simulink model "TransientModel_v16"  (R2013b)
settings: Solver=ode4  StartTime=0.0  StopTime=1500  FixedStep=0.001  RelTol=1e-3
InitFcn:
  | Init_model
StopFcn:
  | Postprocessing2
  | %export_results
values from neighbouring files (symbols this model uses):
  dP = (0:0.005:1)'    [CurveFit_v6_trans.m]
  dP_drag = (0:0.005:1)'    [CurveFit_v6_drag.m]
  Pboost_vec_spd = n_un    [Init_steady_maps.m]
  Pboost_vec_Thr = M_un    [Init_steady_maps.m]
  Pedal = 90    [CurveFit_v6_drag.m]    (also in CurveFit_v6_trans.m = 0:10:90)
  t_sample = 0.01    [Init_model.m]
  time_dy = 0:0.01:5    [CurveFit_v6_drag.m]    (also in CurveFit_v6_trans.m = 0:0.01:10)
undefined symbols (not defined in the file or in its folder): dtaf_sub, dtMbu_sub, dtmf_sub, dtPboost_sub, dtSpeed_Turb_sub, dY, dY_af, dY_af_drag, dY_drag, dY_Mbu, dY_Mbu_drag, dY_mf, dY_mf_drag, dY_Speed_Turb, dY_Speed_Turb_drag, EngineSpeed, EngineSpeed_vec_LM, Mbu_sub_end, Mode, Pboost_Matrix, Speed, Table, Throttle_init, time_dP, time_dP_drag, time_dy_drag, Time_LM, Time_simple, Time_SM, Time_vec_LM
libraries: simulink x45, simulink_extras x4
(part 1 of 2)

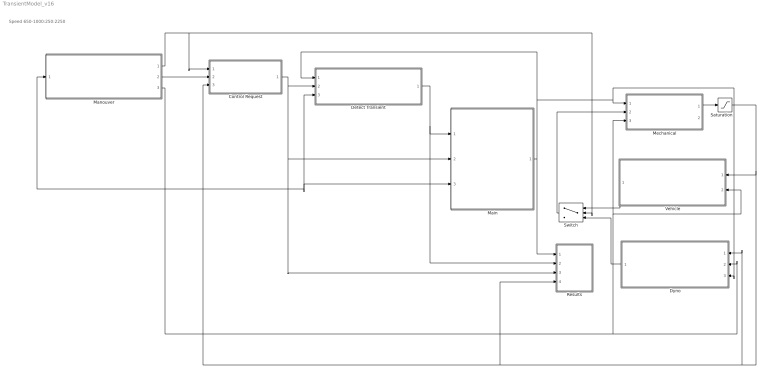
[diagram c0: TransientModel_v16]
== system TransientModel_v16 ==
  note: Speed 650-1000:250:2250
  Control Request : Subsystem
  Detect Transient : Subsystem
  Dyno : Subsystem
  Main : Subsystem
  Manouver : Subsystem
  Mechanical : Subsystem
  Results : Subsystem
  Saturation : Saturate  UpperLimit=2500  LowerLimit=650
  Switch : Switch  Threshold=3
  Vehicle : Subsystem
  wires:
  Mechanical/1(Engine_speed[1/min]) -> Saturation/1
  Switch/1 -> Mechanical/2(Mres[Nm])
  Vehicle/1(Mres[Nm]) -> Switch/1
  Dyno/1(Mdyno[Nm]) -> Switch/3
  Detect Transient/1(BUS_DetectTransient) -> Results/2(BUS_DetectTransient), Main/1(BUS_DetectTransient)
  Main/1(BUS_Main) -> Detect Transient/1(BUS_Main), Dyno/3(BUS_Main), Mechanical/1(BUS_Main), Results/1(BUS_Main)
  Control Request/1(BUS_Requests) -> Detect Transient/2(BUS_Requests), Results/3(BUS_Requests), Main/2(BUS_Requests)
  Saturation/1 -> Vehicle/1(Engine_speed[1/min]), Results/4(Engine_speed), Manouver/1(Engine Speed[1/min]), Control Request/3(Engine_speed[1/min]), Detect Transient/3(Engine_speed), Main/3(Engine Speed[1/min]), Dyno/1(Engine_speed[1/min])
  Manouver/3(Engine_Speed_dem [1/min]) -> Dyno/2(Target_speed[1/min]), Mechanical/3(Engine_speed_init[1/min]), Vehicle/2(Engine_speed_init[1/min])
  Manouver/2(Throttle_position [%]) -> Control Request/2(Throttle_position[%])
  Manouver/1(Mode [-]) -> Control Request/1(Mode[-]), Switch/2

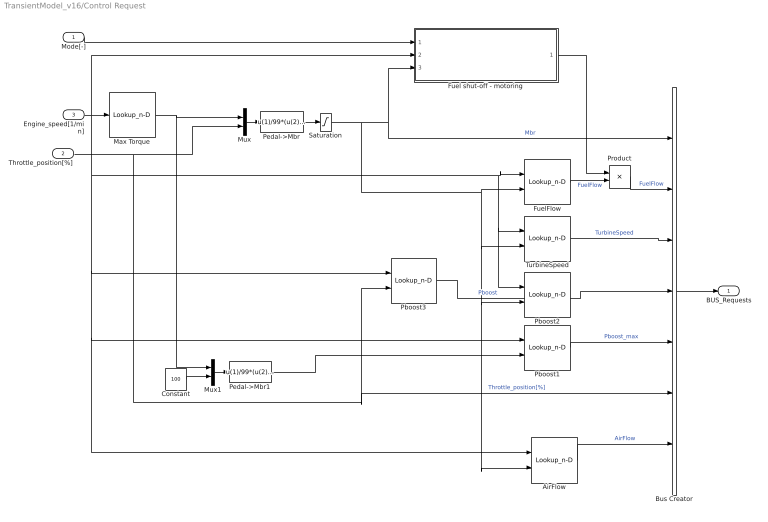
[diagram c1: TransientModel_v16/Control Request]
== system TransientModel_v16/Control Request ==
  Mode[-] : Inport
  Throttle_position[%] : Inport  Port=2
  Engine_speed[1/min] : Inport  Port=3
  AirFlow : Lookup_n-D  BreakpointsForDimension1=Table.Speed  BreakpointsForDimension2=Table.Torque  Table=Table.AirFlow  ExtrapMethod=Clip  UseLastTableValue=on  RndMeth=Simplest
  Bus Creator : BusCreator  Inputs=7
  Constant : Constant  Value=100
  Fuel shut-off - motoring : Subsystem
  FuelFlow : Lookup_n-D  BreakpointsForDimension1=Table.Speed  BreakpointsForDimension2=Table.Torque  Table=Table.FuelFlow  ExtrapMethod=Clip  UseLastTableValue=on  RndMeth=Simplest
  Max Torque : Lookup_n-D  NumberOfTableDimensions=1  BreakpointsForDimension1=|  Table=|  RndMeth=Simplest
      | [650
      | 900
      | 1300
      | 1700
      | 2100
      | 2500
      | ]
      | [400
      | 642.096
      | 868.547
      | 846.784
      | 810.772
      | 701.8]
  Mux : Mux  Inputs=2
  Mux1 : Mux  Inputs=2
  Pboost1 : Lookup_n-D  BreakpointsForDimension1=Table.Speed  BreakpointsForDimension2=Table.Torque  Table=Table.Pboost  ExtrapMethod=Clip  UseLastTableValue=on  RndMeth=Simplest
  Pboost2 : Lookup_n-D  BreakpointsForDimension1=Table.Speed  BreakpointsForDimension2=Table.Torque  Table=Table.Pboost  ExtrapMethod=Clip  UseLastTableValue=on  RndMeth=Simplest
  Pboost3 : Lookup_n-D  BreakpointsForDimension1=Pboost_vec_spd  BreakpointsForDimension2=Pboost_vec_Thr  Table=Pboost_Matrix  ExtrapMethod=Clip  UseLastTableValue=on  RndMeth=Simplest
  Pedal->Mbr : Fcn  Expr=u(1)/99*(u(2)-1)
  Pedal->Mbr1 : Fcn  Expr=u(1)/99*(u(2)-1)
  Product : Product
  Saturation : Saturate  UpperLimit=inf  LowerLimit=0
  TurbineSpeed : Lookup_n-D  BreakpointsForDimension1=Table.Speed  BreakpointsForDimension2=Table.Torque  Table=Table.SpeedTurbine  ExtrapMethod=Clip  UseLastTableValue=on  RndMeth=Simplest
  BUS_Requests : Outport
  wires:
  Mux/1 -> Pedal->Mbr/1
  Throttle_position[%]/1 -> Pboost3/2, Bus Creator/6, Mux/2  "Throttle_position[%]"
  Pedal->Mbr/1 -> Saturation/1
  Mux1/1 -> Pedal->Mbr1/1
  Max Torque/1 -> Mux1/1, Mux/1
  Constant/1 -> Mux1/2
  Pedal->Mbr1/1 -> Pboost1/2
  Pboost1/1 -> Bus Creator/5  "Pboost_max"
  Engine_speed[1/min]/1 -> Fuel shut-off - motoring/2(Engine_speed[1/min]), Max Torque/1, AirFlow/1, Pboost1/1, Pboost3/1, Pboost2/1, TurbineSpeed/1, FuelFlow/1
  Saturation/1 -> AirFlow/2, Pboost2/2, TurbineSpeed/2, FuelFlow/2, Fuel shut-off - motoring/3(Mbr [Nm]), Bus Creator/1  "Mbr"
  Bus Creator/1 -> BUS_Requests/1
  Product/1 -> Bus Creator/2  "FuelFlow"
  TurbineSpeed/1 -> Bus Creator/3  "TurbineSpeed"
  Pboost3/1 -> Bus Creator/4  "Pboost"
  FuelFlow/1 -> Product/2  "FuelFlow"
  AirFlow/1 -> Bus Creator/7  "AirFlow"
  Mode[-]/1 -> Fuel shut-off - motoring/1(Mode[-])
  Fuel shut-off - motoring/1(Fuel shut-off active [-]) -> Product/1

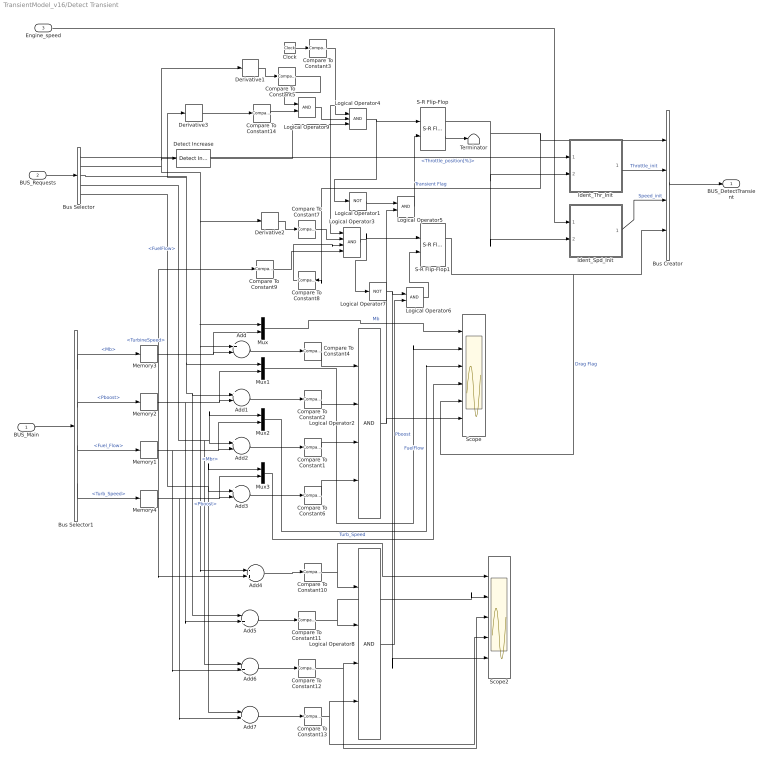
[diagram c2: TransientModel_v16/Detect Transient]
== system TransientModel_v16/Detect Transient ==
  BUS_Main : Inport
  BUS_Requests : Inport  Port=2
  Engine_speed : Inport  Port=3
  Add{,1..3} (4 alike) : Sum  Inputs=+-
  Add{4..7} (4 alike) : Sum  Inputs=-+
  Bus Creator : BusCreator
  Bus Selector : BusSelector  OutputSignals=Throttle_position[%],Mbr,Pboost,FuelFlow,TurbineSpeed
  Bus Selector1 : BusSelector  OutputSignals=Mb,Pboost,Fuel_Flow,Turb_Speed
  Clock : Clock
  Compare To Constant1 : simulink/Logic and Bit Operations/Compare To Constant  relop=<  const=0.01  OutDataTypeStr=boolean
  Compare To Constant10 : simulink/Logic and Bit Operations/Compare To Constant  relop=<  const=5  OutDataTypeStr=boolean
  Compare To Constant11 : simulink/Logic and Bit Operations/Compare To Constant  relop=<  const=0.001  OutDataTypeStr=boolean
  Compare To Constant12 : simulink/Logic and Bit Operations/Compare To Constant  relop=<  const=0.01  OutDataTypeStr=boolean
  Compare To Constant13 : simulink/Logic and Bit Operations/Compare To Constant  relop=<  const=100  OutDataTypeStr=boolean
  Compare To Constant14 : simulink/Logic and Bit Operations/Compare To Constant  relop=>=  const=0.15  OutDataTypeStr=boolean
  Compare To Constant2 : simulink/Logic and Bit Operations/Compare To Constant  relop=<  const=0.001  OutDataTypeStr=boolean
  Compare To Constant3 : simulink/Logic and Bit Operations/Compare To Constant  relop=>=  const=0.1  OutDataTypeStr=boolean
  Compare To Constant4 : simulink/Logic and Bit Operations/Compare To Constant  relop=<  const=5  OutDataTypeStr=boolean
  Compare To Constant5 : simulink/Logic and Bit Operations/Compare To Constant  relop=>=  const=50  OutDataTypeStr=boolean
  Compare To Constant6 : simulink/Logic and Bit Operations/Compare To Constant  relop=<  const=100  OutDataTypeStr=boolean
  Compare To Constant7 : simulink/Logic and Bit Operations/Compare To Constant  relop=<=  const=-50  OutDataTypeStr=boolean
  Compare To Constant8 : simulink/Logic and Bit Operations/Compare To Constant  relop===  const=0  OutDataTypeStr=boolean
  Compare To Constant9 : simulink/Logic and Bit Operations/Compare To Constant  relop=>=  const=50  OutDataTypeStr=boolean
  Derivative1 : Derivative
  Derivative2 : Derivative
  Derivative3 : Derivative
  Detect Increase : simulink/Logic and Bit Operations/Detect Increase  vinit=0.0  InputProcessing=Inherited  OutDataTypeStr=boolean
  Ident_Spd_Init : Subsystem
  Ident_Thr_Init : Subsystem
  Logical Operator1 : Logic  Operator=NOT  AllPortsSameDT=off  OutDataTypeStr=boolean
  Logical Operator2 : Logic  Inputs=4  AllPortsSameDT=off  OutDataTypeStr=boolean
  Logical Operator3 : Logic  Inputs=4  AllPortsSameDT=off  OutDataTypeStr=boolean
  Logical Operator4 : Logic  Inputs=3  AllPortsSameDT=off  OutDataTypeStr=boolean
  Logical Operator5 : Logic  AllPortsSameDT=off  OutDataTypeStr=boolean
  Logical Operator6 : Logic  AllPortsSameDT=off  OutDataTypeStr=boolean
  Logical Operator7 : Logic  Operator=NOT  AllPortsSameDT=off  OutDataTypeStr=boolean
  Logical Operator8 : Logic  Inputs=4  AllPortsSameDT=off  OutDataTypeStr=boolean
  Logical Operator9 : Logic  AllPortsSameDT=off  OutDataTypeStr=boolean
  Memory{1..4} (4 alike) : Memory
  Mux{,1..3} (4 alike) : Mux  Inputs=2
  S-R Flip-Flop : simulink_extras/Flip Flops/S-R Flip-Flop  initial_condition=0
  S-R Flip-Flop1 : simulink_extras/Flip Flops/S-R Flip-Flop  initial_condition=0
  Scope : Scope  NumInputPorts=6
  Scope2 : Scope  NumInputPorts=5
  Terminator : Terminator
  BUS_DetectTransient : Outport
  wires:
  Detect Increase/1 -> Logical Operator4/3
  Add/1 -> Compare To Constant4/1
  Bus Selector1/1 -> Memory3/1  "<Mb>"
  Bus Selector/2 -> Derivative1/1, Detect Increase/1, Mux/1, Add4/1, Add/1, Derivative2/1  "<Mbr>"
  S-R Flip-Flop/1 -> Ident_Spd_Init/2(TransientFlag), Ident_Thr_Init/2(TransientFlag), Compare To Constant8/1, Bus Creator/1  "Transient Flag"
  S-R Flip-Flop/2 -> Terminator/1
  Memory2/1 -> Add5/2, Mux1/2, Add1/2
  Add1/1 -> Compare To Constant2/1
  Bus Selector1/2 -> Memory2/1  "<Pboost>"
  Bus Selector/3 -> Derivative3/1, Add5/1, Add1/1, Mux1/1  "<Pboost>"
  Logical Operator1/1 -> Logical Operator5/1
  Logical Operator5/1 -> S-R Flip-Flop/2
  Memory3/1 -> Add4/2, Compare To Constant9/1, Mux/2, Add/2
  Clock/1 -> Compare To Constant3/1
  Logical Operator4/1 -> Logical Operator1/1, S-R Flip-Flop/1
  Compare To Constant3/1 -> Logical Operator3/1, Logical Operator4/1
  BUS_Requests/1 -> Bus Selector/1
  BUS_Main/1 -> Bus Selector1/1
  Engine_speed/1 -> Ident_Spd_Init/1(Speed)
  Bus Creator/1 -> BUS_DetectTransient/1
  Ident_Thr_Init/1(Throttle_init) -> Bus Creator/2  "Throttle_init"
  Ident_Spd_Init/1(Speed_init) -> Bus Creator/3  "Speed_init"
  Bus Selector/1 -> Ident_Thr_Init/1(Throttle)  "<Throttle_position[%]>"
  Derivative1/1 -> Compare To Constant5/1
  Bus Selector1/3 -> Memory1/1  "<Fuel_Flow>"
  Bus Selector1/4 -> Memory4/1  "<Turb_Speed>"
  Memory1/1 -> Add6/2, Mux2/2, Add2/2
  Memory4/1 -> Add7/2, Mux3/2, Add3/2
  Bus Selector/4 -> Add6/1, Mux2/1, Add2/1  "<FuelFlow>"
  Bus Selector/5 -> Add7/1, Mux3/1, Add3/1  "<TurbineSpeed>"
  Add2/1 -> Compare To Constant1/1
  Add3/1 -> Compare To Constant6/1
  Mux/1 -> Scope/1  "Mb"
  Mux1/1 -> Scope/2  "Pboost"
  Mux2/1 -> Scope/3  "FuelFlow"
  Mux3/1 -> Scope/4  "Turb_Speed"
  Compare To Constant4/1 -> Logical Operator2/1
  Compare To Constant2/1 -> Logical Operator2/2
  Compare To Constant1/1 -> Logical Operator2/3
  Compare To Constant6/1 -> Logical Operator2/4
  Logical Operator2/1 -> Logical Operator5/2, Scope/6
  Derivative2/1 -> Compare To Constant7/1
  Compare To Constant7/1 -> Logical Operator3/2
  Compare To Constant8/1 -> Logical Operator3/3
  Logical Operator3/1 -> S-R Flip-Flop1/1, Logical Operator7/1
  S-R Flip-Flop1/1 -> Scope/5, Bus Creator/4  "Drag Flag"
  Add4/1 -> Compare To Constant10/1
  Logical Operator7/1 -> Scope2/5, Logical Operator6/1
  Logical Operator6/1 -> S-R Flip-Flop1/2
  Add5/1 -> Compare To Constant11/1
  Compare To Constant10/1 -> Scope2/1, Logical Operator8/1
  Compare To Constant11/1 -> Scope2/2, Logical Operator8/2
  Add6/1 -> Compare To Constant12/1
  Compare To Constant12/1 -> Scope2/3, Logical Operator8/3
  Compare To Constant13/1 -> Scope2/4, Logical Operator8/4
  Add7/1 -> Compare To Constant13/1
  Logical Operator8/1 -> Logical Operator6/2
  Compare To Constant9/1 -> Logical Operator3/4
  Derivative3/1 -> Compare To Constant14/1
  Compare To Constant14/1 -> Logical Operator9/2
  Compare To Constant5/1 -> Logical Operator9/1
  Logical Operator9/1 -> Logical Operator4/2

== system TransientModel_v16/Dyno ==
  Engine_speed[1/min] : Inport
  Target_speed[1/min] : Inport  Port=2
  BUS_Main : Inport  Port=3
  Add : Sum  Inputs=-+
  Add1 : Sum
  Bus Selector1 : BusSelector  OutputSignals=Mb
  PID Controller : simulink/Continuous/PID Controller  Controller=PID  TimeDomain=Continuous-time  SampleTime=1  IntegratorMethod=Forward Euler  FilterMethod=Forward Euler  Form=Parallel  P=3  I=0.05  D=0  N=100  InitialConditionSource=internal  InitialConditionForIntegrator=0  InitialConditionForFilter=0  ExternalReset=none  LimitOutput=off  UpperSaturationLimit=1000  LowerSaturationLimit=0  LinearizeAsGain=off  AntiWindupMode=none  Kb=1  TrackingMode=off  Kt=1  PParamMin=[]  PParamMax=[]  IParamMin=[]  IParamMax=[]  DParamMin=[]  DParamMax=[]  NParamMin=[]  NParamMax=[]  KbParamMin=[]  KbParamMax=[]  KtParamMin=[]  KtParamMax=[]  POutMin=[]  POutMax=[]  IOutMin=[]  IOutMax=[]  DOutMin=[]  DOutMax=[]  NOutMin=[]  NOutMax=[]  KbOutMin=[]  KbOutMax=[]  KtOutMin=[]  KtOutMax=[]  IntegratorOutMin=[]  IntegratorOutMax=[]  FilterOutMin=[]  FilterOutMax=[]  SumOutMin=[]  SumOutMax=[]  SumI1OutMin=[]  SumI1OutMax=[]  SumI2OutMin=[]  SumI2OutMax=[]  SumI3OutMin=[]  SumI3OutMax=[]  SumDOutMin=[]  SumDOutMax=[]  SaturationOutMin=[]  SaturationOutMax=[]  IntegratorContinuousStateAttributes=''  IntegratorStateMustResolveToSignalObject=off  IntegratorRTWStateStorageClass=Auto  FilterContinuousStateAttributes=''  FilterStateMustResolveToSignalObject=off  FilterRTWStateStorageClass=Auto
  Mdyno[Nm] : Outport
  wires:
  Target_speed[1/min]/1 -> Add/1
  Add/1 -> PID Controller/1
  PID Controller/1 -> Add1/2
  Engine_speed[1/min]/1 -> Add/2
  Add1/1 -> Mdyno[Nm]/1
  Bus Selector1/1 -> Add1/1  "<Mb>"
  BUS_Main/1 -> Bus Selector1/1

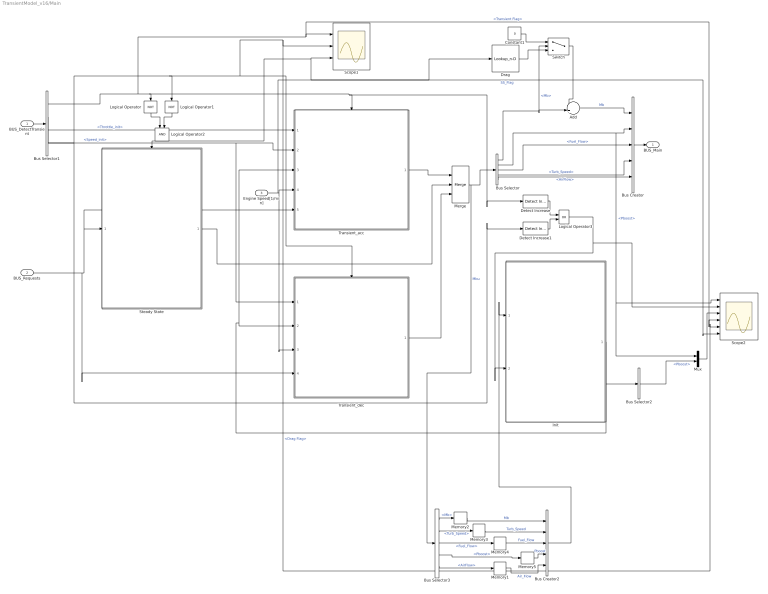
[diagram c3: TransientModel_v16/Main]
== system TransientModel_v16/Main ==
  BUS_DetectTransient : Inport
  BUS_Requests : Inport  Port=2
  Engine Speed[1/min] : Inport  Port=3
  Add : Sum
  Bus Creator : BusCreator  Inputs=5
  Bus Creator2 : BusCreator  Inputs=5
  Bus Selector : BusSelector  OutputSignals=Mb,Pboost,Fuel_Flow,Turb_Speed,AirFlow
  Bus Selector1 : BusSelector  OutputSignals=Transient Flag,Throttle_init,Speed_init,Drag Flag
  Bus Selector2 : BusSelector  OutputSignals=Pboost
  Bus Selector3 : BusSelector  OutputSignals=Mb,Turb_Speed,Fuel_Flow,Pboost,AirFlow
  Constant1 : Constant  Value=0
  Detect Increase : simulink/Logic and Bit Operations/Detect Increase  vinit=0.0  InputProcessing=Inherited  OutDataTypeStr=boolean
  Detect Increase1 : simulink/Logic and Bit Operations/Detect Increase  vinit=0.0  InputProcessing=Inherited  OutDataTypeStr=boolean
  Drag : Lookup_n-D  NumberOfTableDimensions=1  BreakpointsForDimension1="[650\t900\t1000\t1250\t1500\t1750\t2000\t2250]"  Table="[-51.7357\t-47.0411\t-45.0088\t-41.7046\t-40.0756\t-40.1524\t-41.9488\t-44.625 ]"  InternalRulePriority=Speed  RndMeth=Simplest
  Init : Subsystem  TreatAsAtomicUnit=on
  Logical Operator : Logic  Operator=NOT  AllPortsSameDT=off  OutDataTypeStr=boolean
  Logical Operator1 : Logic  Operator=NOT  AllPortsSameDT=off  OutDataTypeStr=boolean
  Logical Operator2 : Logic  AllPortsSameDT=off  OutDataTypeStr=boolean
  Logical Operator3 : Logic  Operator=OR  AllPortsSameDT=off  OutDataTypeStr=boolean
  Memory1 : Memory  X0=1
  Memory2 : Memory
  Memory3 : Memory
  Memory4 : Memory
  Memory5 : Memory  X0=1
  Merge : Merge  Inputs=3
  Mux : Mux  Inputs=2
  Scope1 : Scope  NumInputPorts=3
  Scope2 : Scope  NumInputPorts=6
  Steady State : Subsystem  TreatAsAtomicUnit=on
  Switch : Switch  Threshold=-20
  Transient_acc : Subsystem  TreatAsAtomicUnit=on
  Transient_dec : Subsystem  TreatAsAtomicUnit=on
  BUS_Main : Outport
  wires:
  Engine Speed[1/min]/1 -> Drag/1, Transient_dec/3(Speed), Transient_acc/4(Speed)
  Transient_acc/1(BUS_Transient) -> Merge/1
  Steady State/1(BUS_SS) -> Merge/2
  Merge/1 -> Bus Selector3/1, Bus Selector/1  "Mbu"
  Bus Selector/1 -> Switch/2, Add/2  "<Mb>"
  Bus Creator/1 -> BUS_Main/1
  Bus Selector/3 -> Bus Creator/3  "<Fuel_Flow>"
  Bus Selector/2 -> Scope2/1, Mux/1, Bus Creator/2  "<Pboost>"
  Bus Selector/4 -> Bus Creator/4  "<Turb_Speed>"
  BUS_Requests/1 -> Transient_dec/4(BUS_Requests), Steady State/1(BUS_Requests), Transient_acc/5(BUS_Requests)
  BUS_DetectTransient/1 -> Bus Selector1/1
  Bus Selector1/1 -> Scope2/4, Scope1/1, Detect Increase/1, Transient_acc/Enable, Logical Operator/1  "<Transient Flag>"
  Bus Selector1/2 -> Transient_acc/1(Throttle[%])  "<Throttle_init>"
  Bus Selector1/3 -> Transient_dec/1(Speed_init), Transient_acc/2(Speed_init)  "<Speed_init>"
  Bus Selector1/4 -> Detect Increase1/1, Logical Operator1/1, Scope2/5, Scope1/2, Transient_dec/Enable  "<Drag Flag>"
  Transient_dec/1(BUS_Transient) -> Merge/3
  Logical Operator1/1 -> Logical Operator2/2
  Logical Operator/1 -> Logical Operator2/1
  Logical Operator2/1 -> Steady State/Enable, Scope2/6, Scope1/3  "SS_Flag"
  Detect Increase/1 -> Logical Operator3/1
  Detect Increase1/1 -> Logical Operator3/2
  Logical Operator3/1 -> Init/2(Enable), Scope2/2
  Mux/1 -> Scope2/3
  Bus Selector3/1 -> Memory2/1  "<Mb>"
  Bus Selector3/2 -> Memory3/1  "<Turb_Speed>"
  Bus Selector3/3 -> Memory4/1  "<Fuel_Flow>"
  Bus Selector3/4 -> Memory5/1  "<Pboost>"
  Memory2/1 -> Bus Creator2/1  "Mb"
  Memory3/1 -> Bus Creator2/2  "Turb_Speed"
  Memory4/1 -> Bus Creator2/3  "Fuel_Flow"
  Memory5/1 -> Bus Creator2/4  "Pboost"
  Bus Creator2/1 -> Init/1(BUS_Requests)
  Init/1(BUS_init) -> Bus Selector2/1, Transient_dec/2(BUS_init), Transient_acc/3(BUS_init)
  Bus Selector2/1 -> Mux/2  "<Pboost>"
  Constant1/1 -> Switch/1
  Drag/1 -> Switch/3
  Add/1 -> Bus Creator/1  "Mb"
  Switch/1 -> Add/1
  Bus Selector3/5 -> Memory1/1  "<AirFlow>"
  Memory1/1 -> Bus Creator2/5  "Air_Flow"
  Bus Selector/5 -> Bus Creator/5  "<AirFlow>"

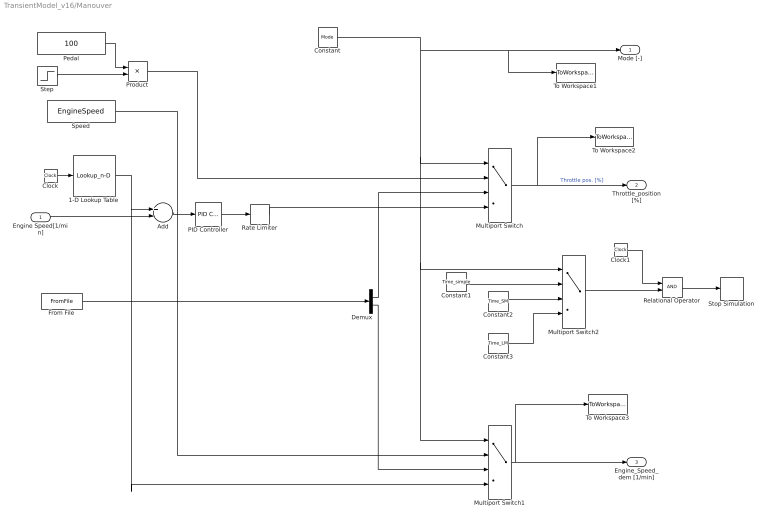
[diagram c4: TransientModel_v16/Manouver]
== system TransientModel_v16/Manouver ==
  Engine Speed[1/min] : Inport
  1-D Lookup Table : Lookup_n-D  NumberOfTableDimensions=1  BreakpointsForDimension1=Time_vec_LM  Table=EngineSpeed_vec_LM  InternalRulePriority=Speed  RndMeth=Simplest
  Add : Sum  Inputs=+-
  Clock : Clock
  Clock1 : Clock
  Constant : Constant  Value=Mode
  Constant1 : Constant  Value=Time_simple
  Constant2 : Constant  Value=Time_SM
  Constant3 : Constant  Value=Time_LM
  Demux : Demux  Outputs=2
  From File : FromFile  FileName=WHTC.mat  SampleTime=0
  Multiport Switch : MultiPortSwitch
  Multiport Switch1 : MultiPortSwitch
  Multiport Switch2 : MultiPortSwitch
  PID Controller : simulink/Continuous/PID Controller  Controller=PID  TimeDomain=Continuous-time  SampleTime=1  IntegratorMethod=Forward Euler  FilterMethod=Forward Euler  Form=Parallel  P=1  I=0.3  D=0  N=100  InitialConditionSource=internal  InitialConditionForIntegrator=25  InitialConditionForFilter=0  ExternalReset=none  LimitOutput=on  UpperSaturationLimit=100  LowerSaturationLimit=0  LinearizeAsGain=off  AntiWindupMode=clamping  Kb=1  TrackingMode=off  Kt=1  PParamMin=[]  PParamMax=[]  IParamMin=[]  IParamMax=[]  DParamMin=[]  DParamMax=[]  NParamMin=[]  NParamMax=[]  KbParamMin=[]  KbParamMax=[]  KtParamMin=[]  KtParamMax=[]  POutMin=[]  POutMax=[]  IOutMin=[]  IOutMax=[]  DOutMin=[]  DOutMax=[]  NOutMin=[]  NOutMax=[]  KbOutMin=[]  KbOutMax=[]  KtOutMin=[]  KtOutMax=[]  IntegratorOutMin=[]  IntegratorOutMax=[]  FilterOutMin=[]  FilterOutMax=[]  SumOutMin=[]  SumOutMax=[]  SumI1OutMin=[]  SumI1OutMax=[]  SumI2OutMin=[]  SumI2OutMax=[]  SumI3OutMin=[]  SumI3OutMax=[]  SumDOutMin=[]  SumDOutMax=[]  SaturationOutMin=[]  SaturationOutMax=[]  IntegratorContinuousStateAttributes=''  IntegratorStateMustResolveToSignalObject=off  IntegratorRTWStateStorageClass=Auto  FilterContinuousStateAttributes=''  FilterStateMustResolveToSignalObject=off  FilterRTWStateStorageClass=Auto
  Pedal : Constant  Value=100
  Product : Product
  Rate Limiter : RateLimiter  RisingSlewLimit=inf  FallingSlewLimit=-200  SampleTimeMode=inherited
  Relational Operator : RelationalOperator  OutDataTypeStr=boolean
  Speed : Constant  Value=EngineSpeed
  Step : Step  Time=5  Before=Throttle_init/100  SampleTime=0
  Stop Simulation : Stop
  To Workspace1 : ToWorkspace  VariableName=Mode  SampleTime=-1
  To Workspace2 : ToWorkspace  VariableName=Pedal_set  SampleTime=-1
  To Workspace3 : ToWorkspace  VariableName=Speed_set  SampleTime=-1
  Mode [-] : Outport
  Throttle_position [%] : Outport  Port=2
  Engine_Speed_dem [1/min] : Outport  Port=3
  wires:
  Step/1 -> Product/2
  Pedal/1 -> Product/1
  Multiport Switch1/1 -> Engine_Speed_dem [1/min]/1, To Workspace3/1
  From File/1 -> Demux/1
  Demux/1 -> Multiport Switch/3
  Demux/2 -> Multiport Switch1/3
  Add/1 -> PID Controller/1
  Clock/1 -> 1-D Lookup Table/1
  1-D Lookup Table/1 -> Multiport Switch1/4, Add/1
  PID Controller/1 -> Rate Limiter/1
  Engine Speed[1/min]/1 -> Add/2
  Product/1 -> Multiport Switch/2
  Rate Limiter/1 -> Multiport Switch/4
  Speed/1 -> Multiport Switch1/2
  Multiport Switch/1 -> Throttle_position [%]/1, To Workspace2/1  "Throttle pos. [%]"
  Constant/1 -> To Workspace1/1, Mode [-]/1, Multiport Switch/1, Multiport Switch1/1, Multiport Switch2/1
  Constant1/1 -> Multiport Switch2/2
  Constant2/1 -> Multiport Switch2/3
  Constant3/1 -> Multiport Switch2/4
  Clock1/1 -> Relational Operator/1
  Multiport Switch2/1 -> Relational Operator/2
  Relational Operator/1 -> Stop Simulation/1

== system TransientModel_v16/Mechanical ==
  BUS_Main : Inport
  Mres[Nm] : Inport  Port=2
  Engine_speed_init[1/min] : Inport  Port=3
  Add1 : Sum  Inputs=+-
  Bus Selector1 : BusSelector  OutputSignals=Mb
  Gain : Gain  Gain=1/1.2
  Gain1 : Gain  Gain=pi/30
  Integrator : Integrator  InitialConditionSource=external  InitialCondition=2000/30*pi
  Product : Product
  rad2rpm1 : Gain  Gain=30/pi
  Engine_speed[1/min] : Outport
  Pemech : Outport  Port=2
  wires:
  Product/1 -> Pemech/1
  Integrator/1 -> Product/1, rad2rpm1/1  "om_e"
  Gain/1 -> Integrator/1
  Add1/1 -> Gain/1
  rad2rpm1/1 -> Engine_speed[1/min]/1
  Mres[Nm]/1 -> Add1/2
  Engine_speed_init[1/min]/1 -> Gain1/1
  Gain1/1 -> Integrator/2
  Bus Selector1/1 -> Add1/1, Product/2  "<Mb>"
  BUS_Main/1 -> Bus Selector1/1

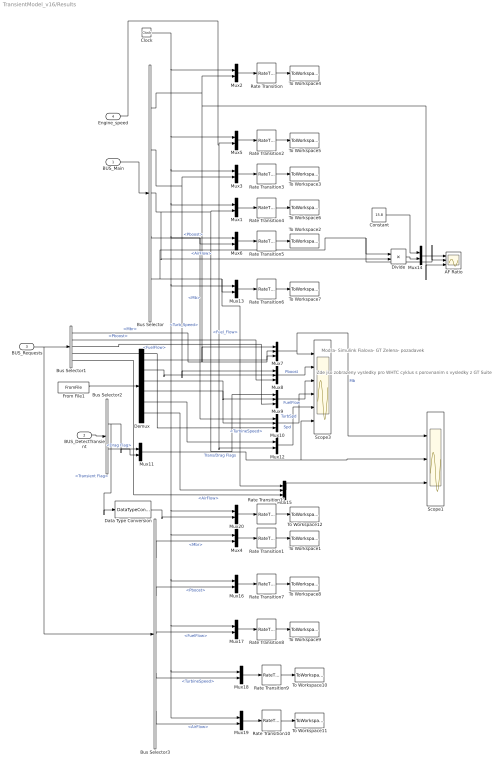
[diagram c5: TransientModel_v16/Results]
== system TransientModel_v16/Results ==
  note: Zde jso zobrazeny vysledky pro WHTC cyklus s porovnanim s vysledky z GT Suite
  note: Modra- Simulink Fialova- GT Zelena- pozadavek
  BUS_Main : Inport
  BUS_DetectTransient : Inport  Port=2
  BUS_Requests : Inport  Port=3
  Engine_speed : Inport  Port=4
  AF Ratio : Scope  NumInputPorts=3
  Bus Selector : BusSelector  OutputSignals=Mb,Pboost,Fuel_Flow,Turb_Speed,AirFlow
  Bus Selector1 : BusSelector  OutputSignals=Mbr,Pboost,FuelFlow,TurbineSpeed,AirFlow
  Bus Selector2 : BusSelector  OutputSignals=Transient Flag,Drag Flag
  Bus Selector3 : BusSelector  OutputSignals=Mbr,Pboost,FuelFlow,TurbineSpeed,AirFlow
  Clock : Clock
  Constant : Constant  Value=15.8
  Data Type Conversion : DataTypeConversion
  Demux : Demux  Outputs=6
  Divide : Product  Inputs=*/
  From File1 : FromFile  FileName=GT_WHTC_speed2.mat  SampleTime=0
  Mux{1..6,11..14,16..20} (15 alike) : Mux  Inputs=2
  Mux{7..10,15} (5 alike) : Mux  Inputs=3
  Rate Transition{,1..11} (12 alike) : RateTransition
  Scope1 : Scope  NumInputPorts=3
  Scope3 : Scope  NumInputPorts=6
  To Workspace1 : ToWorkspace  VariableName=Sim2GT_Mbr  SampleTime=t_sample
  To Workspace10 : ToWorkspace  VariableName=Sim2GT_TurbSpeed_r  SampleTime=t_sample
  To Workspace11 : ToWorkspace  VariableName=Sim2GT_AirFlow_r  SampleTime=t_sample
  To Workspace12 : ToWorkspace  VariableName=Sim2GT_Trans_Flag  SampleTime=t_sample
  To Workspace2 : ToWorkspace  VariableName=Sim2GT_TurbSpeed  SampleTime=t_sample
  To Workspace3 : ToWorkspace  VariableName=Sim2GT_Pboost  SampleTime=t_sample
  To Workspace4 : ToWorkspace  VariableName=Sim2GT_Mb  SampleTime=t_sample
  To Workspace5 : ToWorkspace  VariableName=Sim2GT_speed  SampleTime=t_sample
  To Workspace6 : ToWorkspace  VariableName=Sim2GT_Mb_FuelFlow  SampleTime=t_sample
  To Workspace7 : ToWorkspace  VariableName=Sim2GT_AirFlow  SampleTime=t_sample
  To Workspace8 : ToWorkspace  VariableName=Sim2GT_Pboost_r  SampleTime=t_sample
  To Workspace9 : ToWorkspace  VariableName=Sim2GT_Mb_FuelFlow_r  SampleTime=t_sample
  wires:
  Rate Transition/1 -> To Workspace4/1
  Mux2/1 -> Rate Transition/1
  Rate Transition2/1 -> To Workspace5/1
  Mux5/1 -> Rate Transition2/1
  Rate Transition3/1 -> To Workspace3/1
  Mux3/1 -> Rate Transition3/1
  Bus Selector1/1 -> Mux7/3  "<Mbr>"
  Engine_speed/1 -> Mux12/2, Mux5/2
  Bus Selector/2 -> Mux8/1, Mux3/2  "<Pboost>"
  BUS_Main/1 -> Bus Selector/1
  Bus Selector/1 -> AF Ratio/3, Mux7/1, Mux2/2  "<Mb>"
  Clock/1 -> Mux2/1, Mux5/1, Mux19/1, Mux18/1, Mux17/1, Mux16/1, Mux4/1, Mux20/1, Mux13/1, Mux6/1, Mux1/1, Mux3/1
  Rate Transition4/1 -> To Workspace6/1
  Mux1/1 -> Rate Transition4/1
  Rate Transition5/1 -> To Workspace2/1
  Mux6/1 -> Rate Transition5/1
  Bus Selector/4 -> Mux10/1, Mux6/2  "<Turb_Speed>"
  Bus Selector/3 -> Divide/2, Mux9/1, Mux1/2  "<Fuel_Flow>"
  From File1/1 -> Demux/1
  Demux/1 -> Mux7/2
  Mux7/1 -> Scope1/1, Scope3/1  "Mb"
  Mux8/1 -> Scope3/2  "Pboost"
  Mux9/1 -> Scope3/3  "FuelFlow"
  Mux10/1 -> Scope3/4  "TurbSpd"
  Demux/2 -> Mux8/2
  Demux/3 -> Mux9/2
  Demux/4 -> Mux10/2
  Bus Selector1/2 -> Mux8/3  "<Pboost>"
  BUS_Requests/1 -> Bus Selector3/1, Bus Selector1/1
  BUS_DetectTransient/1 -> Bus Selector2/1
  Bus Selector2/1 -> Data Type Conversion/1, Mux11/1  "<Transient Flag>"
  Bus Selector2/2 -> Mux11/2  "<Drag Flag>"
  Demux/5 -> Mux12/1
  Mux12/1 -> Scope3/5  "Spd"
  Mux11/1 -> Scope1/2, Scope3/6  "Trans/Drag Flags"
  Bus Selector1/3 -> Mux9/3  "<FuelFlow>"
  Bus Selector1/4 -> Mux10/3  "<TurbineSpeed>"
  Bus Selector/5 -> AF Ratio/2, Divide/1, Mux15/1, Mux13/2  "<AirFlow>"
  Mux13/1 -> Rate Transition6/1
  Rate Transition6/1 -> To Workspace7/1
  Mux14/1 -> AF Ratio/1
  Divide/1 -> Mux14/2
  Constant/1 -> Mux14/1
  Demux/6 -> Mux15/2
  Bus Selector1/5 -> Mux15/3  "<AirFlow>"
  Mux15/1 -> Scope1/3
  Rate Transition7/1 -> To Workspace8/1
  Mux16/1 -> Rate Transition7/1
  Bus Selector3/2 -> Mux16/2  "<Pboost>"
  Rate Transition8/1 -> To Workspace9/1
  Mux17/1 -> Rate Transition8/1
  Bus Selector3/3 -> Mux17/2  "<FuelFlow>"
  Rate Transition9/1 -> To Workspace10/1
  Mux18/1 -> Rate Transition9/1
  Bus Selector3/4 -> Mux18/2  "<TurbineSpeed>"
  Rate Transition1/1 -> To Workspace1/1
  Mux4/1 -> Rate Transition1/1
  Bus Selector3/1 -> Mux4/2  "<Mbr>"
  Mux19/1 -> Rate Transition10/1
  Rate Transition10/1 -> To Workspace11/1
  Bus Selector3/5 -> Mux19/2  "<AirFlow>"
  Rate Transition11/1 -> To Workspace12/1
  Mux20/1 -> Rate Transition11/1
  Data Type Conversion/1 -> Mux20/2

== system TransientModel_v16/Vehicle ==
  Engine_speed[1/min] : Inport
  Engine_speed_init[1/min] : Inport  Port=2
  Add4 : Sum  Inputs=+-
  Add5 : Sum
  Driving resistance : Lookup_n-D  NumberOfTableDimensions=1  BreakpointsForDimension1=|  Table=|  ExtrapMethod=Clip  RndMeth=Simplest
      | [650
      | 900
      | 1000
      | 1100
      | 1200
      | 1300
      | 1400
      | 1500
      | 1600
      | 1700
      | 1800
      | 1900
      | 2000
      | 2100
      | 2200
      | 2300
      | 2400
      | 2500
      | 2600
      | 2700]
      | [140.201383
      | 153.6645939
      | 160.2659102
      | 167.5621018
      | 175.5531689
      | 184.2391114
      | 193.6199293
      | 203.6956225
      | 214.4661912
      | 225.9316353
      | 238.0919548
      | 250.9471496
      | 264.4972199
      | 278.7421655
      | 293.6819866
      | 309.3166831
      | 325.6462549
      | 342.6707022
      | 360.3900248
      | 378.8042229]
  Gain1 : Gain  Gain=pi/30
  Idle_gear & Blocker Ring : Gain  Gain=1/74.4
  Integrator1 : Integrator  InitialConditionSource=external  InitialCondition=900/30*pi
  Integrator3 : Integrator
  Sum : Sum  Inputs=+-
  b_cg : Gain  Gain=5
  k_cg : Gain  Gain=2500000
  n2rad : Gain  Gain=pi/30
  rad2rpm : Gain  Gain=30/pi
  Mres[Nm] : Outport
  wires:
  b_cg/1 -> Add5/2
  k_cg/1 -> Add5/1
  Integrator3/1 -> k_cg/1
  Add4/1 -> Integrator3/1, b_cg/1
  Idle_gear & Blocker Ring/1 -> Integrator1/1
  Sum/1 -> Idle_gear & Blocker Ring/1
  Integrator1/1 -> rad2rpm/1, Add4/2
  rad2rpm/1 -> Driving resistance/1
  Engine_speed[1/min]/1 -> n2rad/1
  n2rad/1 -> Add4/1
  Driving resistance/1 -> Sum/2
  Add5/1 -> Mres[Nm]/1, Sum/1
  Engine_speed_init[1/min]/1 -> Gain1/1
  Gain1/1 -> Integrator1/2

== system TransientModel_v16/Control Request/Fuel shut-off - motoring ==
  Mode[-] : Inport
  Engine_speed[1/min] : Inport  Port=2
  Mbr [Nm] : Inport  Port=3
  0 : Constant  Value=0
  1 : Constant
  Compare To Constant : simulink/Logic and Bit Operations/Compare To Constant  relop=<=  const=0  OutDataTypeStr=boolean
  Fuel-shut-off : Switch  Threshold=3
  Fuel-shut-off rpm : simulink/Logic and Bit Operations/Compare To Constant  relop=>=  const=900  OutDataTypeStr=boolean
  Logical Operator : Logic  Operator=NAND  Inputs=3  AllPortsSameDT=off  OutDataTypeStr=boolean
  Fuel shut-off active [-] : Outport
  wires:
  Compare To Constant/1 -> Logical Operator/1
  Fuel-shut-off rpm/1 -> Logical Operator/2
  Logical Operator/1 -> Fuel shut-off active [-]/1
  Fuel-shut-off/1 -> Logical Operator/3
  Mbr [Nm]/1 -> Compare To Constant/1
  Engine_speed[1/min]/1 -> Fuel-shut-off rpm/1
  1/1 -> Fuel-shut-off/1
  0/1 -> Fuel-shut-off/3
  Mode[-]/1 -> Fuel-shut-off/2

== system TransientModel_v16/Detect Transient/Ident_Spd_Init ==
  Speed : Inport
  TransientFlag : Inport  Port=2
  Clock : Clock
  Compare To Constant : simulink/Logic and Bit Operations/Compare To Constant  relop=>=  const=0.1  OutDataTypeStr=uint8
  Detect Increase : simulink/Logic and Bit Operations/Detect Increase  vinit=0.0  InputProcessing=Inherited  OutDataTypeStr=uint8
  Enabled Subsystem : Subsystem  TreatAsAtomicUnit=on
  Logical Operator : Logic  AllPortsSameDT=off  OutDataTypeStr=boolean
  Memory : Memory
  Memory1 : Memory
  S-R Flip-Flop : simulink_extras/Flip Flops/S-R Flip-Flop  initial_condition=0
  Switch : Switch
  Speed_init : Outport
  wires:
  TransientFlag/1 -> Detect Increase/1
  Memory1/1 -> Enabled Subsystem/1(In1)
  Memory/1 -> Switch/1
  Enabled Subsystem/1(Out1) -> Switch/3
  Switch/1 -> Speed_init/1, Memory1/1
  Compare To Constant/1 -> Logical Operator/2
  Clock/1 -> Compare To Constant/1
  Logical Operator/1 -> Switch/2, S-R Flip-Flop/1
  Detect Increase/1 -> Logical Operator/1
  S-R Flip-Flop/1 -> Enabled Subsystem/Enable
  Speed/1 -> Memory/1

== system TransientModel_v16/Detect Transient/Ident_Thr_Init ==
  Throttle : Inport
  TransientFlag : Inport  Port=2
  Clock : Clock
  Compare To Constant : simulink/Logic and Bit Operations/Compare To Constant  relop=>=  const=0.1  OutDataTypeStr=uint8
  Detect Increase : simulink/Logic and Bit Operations/Detect Increase  vinit=0.0  InputProcessing=Inherited  OutDataTypeStr=uint8
  Enabled Subsystem : Subsystem  TreatAsAtomicUnit=on
  Logical Operator : Logic  AllPortsSameDT=off  OutDataTypeStr=boolean
  Memory : Memory
  Memory1 : Memory
  S-R Flip-Flop : simulink_extras/Flip Flops/S-R Flip-Flop  initial_condition=0
  Switch : Switch
  Throttle_init : Outport
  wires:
  Throttle/1 -> Memory/1
  S-R Flip-Flop/1 -> Enabled Subsystem/Enable
  Detect Increase/1 -> Logical Operator/1
  Logical Operator/1 -> S-R Flip-Flop/1, Switch/2
  Clock/1 -> Compare To Constant/1
  Compare To Constant/1 -> Logical Operator/2
  Switch/1 -> Memory1/1, Throttle_init/1
  Enabled Subsystem/1(Out1) -> Switch/3
  Memory/1 -> Switch/1
  Memory1/1 -> Enabled Subsystem/1(In1)
  TransientFlag/1 -> Detect Increase/1

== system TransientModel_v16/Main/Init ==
  BUS_Requests : Inport
  Enable : Inport  Port=2
  Subsystem : Subsystem
  BUS_init : Outport
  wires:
  BUS_Requests/1 -> Subsystem/1(In1)
  Enable/1 -> Subsystem/Enable
  Subsystem/1(Out1) -> BUS_init/1

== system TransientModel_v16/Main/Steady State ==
  BUS_Requests : Inport
  Enable : EnablePort
  Bus Creator1 : BusCreator  Inputs=5
  Bus Selector : BusSelector  OutputSignals=Mbr,TurbineSpeed,FuelFlow,Pboost,AirFlow
  Gain{,1..4} (5 alike) : Gain
  Memory{1..5} (5 alike) : Memory
  BUS_SS : Outport
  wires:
  Bus Selector/2 -> Memory3/1, Gain1/1  "<TurbineSpeed>"
  Bus Selector/3 -> Gain2/1, Memory1/1  "<FuelFlow>"
  Bus Selector/4 -> Gain3/1, Memory4/1  "<Pboost>"
  Bus Creator1/1 -> BUS_SS/1
  Gain/1 -> Bus Creator1/2  "Mb"
  Gain3/1 -> Bus Creator1/1  "Pboost"
  Gain2/1 -> Bus Creator1/3  "Fuel_Flow"
  Gain1/1 -> Bus Creator1/4  "Turb_Speed"
  BUS_Requests/1 -> Bus Selector/1
  Bus Selector/1 -> Memory2/1, Gain/1  "<Mbr>"
  Bus Selector/5 -> Memory5/1, Gain4/1  "<AirFlow>"
  Gain4/1 -> Bus Creator1/5  "AirFlow"

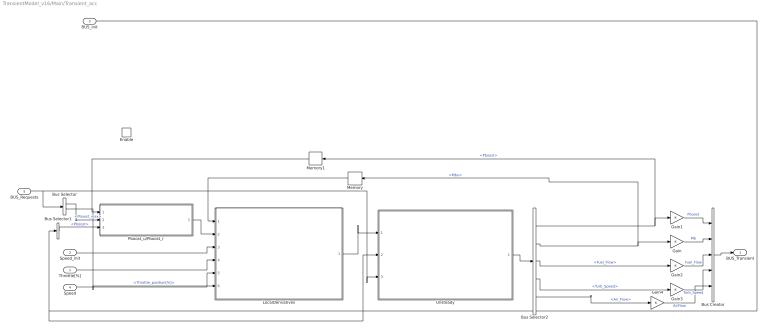
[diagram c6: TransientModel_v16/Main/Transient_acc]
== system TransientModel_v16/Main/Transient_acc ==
  Throttle[%] : Inport
  Speed_init : Inport  Port=2
  BUS_init : Inport  Port=3
  Speed : Inport  Port=4
  BUS_Requests : Inport  Port=5
  Enable : EnablePort  StatesWhenEnabling=reset
  Bus Creator : BusCreator  Inputs=5
  Bus Selector : BusSelector  OutputSignals=Pboost_max,Throttle_position[%]
  Bus Selector1 : BusSelector  OutputSignals=Pboost
  Bus Selector2 : BusSelector  OutputSignals=Pboost,Mbu,Fuel_Flow,Turb_Speed,Air_Flow
  Gain{,1..4} (5 alike) : Gain
  LocalDerivatives : Subsystem
  Memory : Memory
  Memory1 : Memory
  Pboost_u/Pboost_r : Subsystem
  Unsteady : Subsystem
  BUS_Transient : Outport
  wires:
  Bus Creator/1 -> BUS_Transient/1
  Gain1/1 -> Bus Creator/1  "Pboost"
  Gain/1 -> Bus Creator/2  "Mb"
  Gain2/1 -> Bus Creator/3  "Fuel_Flow"
  Gain3/1 -> Bus Creator/4  "Turb_Speed"
  Speed/1 -> LocalDerivatives/5(Speed)
  Speed_init/1 -> LocalDerivatives/3(Speed_init)
  Throttle[%]/1 -> LocalDerivatives/4(Throttle_init[%])
  Pboost_u/Pboost_r/1(Pboost_u/Pboost_r) -> LocalDerivatives/2(Pboost_u/Pboost_r)
  Bus Selector1/1 -> Pboost_u/Pboost_r/3(Pboost_init)  "<Pboost>"
  LocalDerivatives/1(BUS_Derivatives) -> Unsteady/1(BUS_Derivatives)
  Unsteady/1(BUS_Unsteady) -> Bus Selector2/1
  Bus Selector2/2 -> Memory/1, Gain/1  "<Mbu>"
  Bus Selector2/1 -> Memory1/1, Gain1/1  "<Pboost>"
  Bus Selector2/3 -> Gain2/1  "<Fuel_Flow>"
  Bus Selector2/4 -> Gain3/1  "<Turb_Speed>"
  Memory/1 -> LocalDerivatives/1(Mbu)
  Memory1/1 -> Pboost_u/Pboost_r/1(Pboost_u)
  BUS_Requests/1 -> Bus Selector/1, Unsteady/3(BUS_Requests)
  Bus Selector/1 -> Pboost_u/Pboost_r/2(Pboostr_max[bar])  "<Pboost_max>"
  BUS_init/1 -> Bus Selector1/1, Unsteady/2(BUS_init)
  Gain4/1 -> Bus Creator/5  "AirFlow"
  Bus Selector2/5 -> Gain4/1  "<Air_Flow>"
  Bus Selector/2 -> LocalDerivatives/6(Throttle_act[%])  "<Throttle_position[%]>"

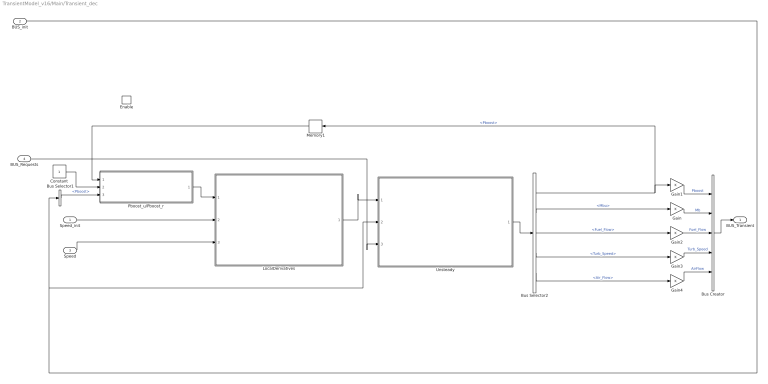
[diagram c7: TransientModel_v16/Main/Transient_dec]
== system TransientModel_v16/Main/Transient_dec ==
  Speed_init : Inport
  BUS_init : Inport  Port=2
  Speed : Inport  Port=3
  BUS_Requests : Inport  Port=4
  Enable : EnablePort  StatesWhenEnabling=reset
  Bus Creator : BusCreator  Inputs=5
  Bus Selector1 : BusSelector  OutputSignals=Pboost
  Bus Selector2 : BusSelector  OutputSignals=Pboost,Mbu,Fuel_Flow,Turb_Speed,Air_Flow
  Constant : Constant
  Gain{,1..4} (5 alike) : Gain
  LocalDerivatives : Subsystem
  Memory1 : Memory
  Pboost_u/Pboost_r : Subsystem
  Unsteady : Subsystem
  BUS_Transient : Outport
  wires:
  BUS_Requests/1 -> Unsteady/3(BUS_Requests)
  Memory1/1 -> Pboost_u/Pboost_r/1(Pboost_u)
  Bus Selector2/4 -> Gain3/1  "<Turb_Speed>"
  Bus Selector2/3 -> Gain2/1  "<Fuel_Flow>"
  Bus Selector2/1 -> Gain1/1, Memory1/1  "<Pboost>"
  Bus Selector2/2 -> Gain/1  "<Mbu>"
  Unsteady/1(BUS_Unsteady) -> Bus Selector2/1
  LocalDerivatives/1(BUS_Derivatives) -> Unsteady/1(BUS_Derivatives)
  Bus Selector1/1 -> Pboost_u/Pboost_r/3(Pboost_init)  "<Pboost>"
  Pboost_u/Pboost_r/1(Pboost_u/Pboost_r) -> LocalDerivatives/1(Pboost_u/Pboost_r)
  Speed_init/1 -> LocalDerivatives/2(Speed_init)
  Speed/1 -> LocalDerivatives/3(Speed)
  Gain3/1 -> Bus Creator/4  "Turb_Speed"
  Gain2/1 -> Bus Creator/3  "Fuel_Flow"
  Gain/1 -> Bus Creator/2  "Mb"
  Gain1/1 -> Bus Creator/1  "Pboost"
  BUS_init/1 -> Bus Selector1/1, Unsteady/2(BUS_init)
  Bus Creator/1 -> BUS_Transient/1
  Constant/1 -> Pboost_u/Pboost_r/2(Pboostr_max[bar])
  Gain4/1 -> Bus Creator/5  "AirFlow"
  Bus Selector2/5 -> Gain4/1  "<Air_Flow>"

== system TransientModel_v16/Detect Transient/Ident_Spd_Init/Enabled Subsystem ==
  In1 : Inport
  Enable : EnablePort
  Out1 : Outport
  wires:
  In1/1 -> Out1/1

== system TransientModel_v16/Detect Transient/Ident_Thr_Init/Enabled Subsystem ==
  In1 : Inport
  Enable : EnablePort
  Out1 : Outport
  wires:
  In1/1 -> Out1/1

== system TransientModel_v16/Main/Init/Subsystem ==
  In1 : Inport
  Enable : EnablePort
  Bus Creator2 : BusCreator  Inputs=5
  Bus Selector : BusSelector  OutputSignals=Mb,Turb_Speed,Fuel_Flow,Pboost,Air_Flow
  Out1 : Outport
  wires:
  In1/1 -> Bus Selector/1
  Bus Selector/1 -> Bus Creator2/1  "<Mb>"
  Bus Selector/2 -> Bus Creator2/2  "<Turb_Speed>"
  Bus Selector/3 -> Bus Creator2/3  "<Fuel_Flow>"
  Bus Selector/4 -> Bus Creator2/4  "<Pboost>"
  Bus Creator2/1 -> Out1/1
  Bus Selector/5 -> Bus Creator2/5  "<Air_Flow>"

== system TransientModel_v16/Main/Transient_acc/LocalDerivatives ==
  Mbu : Inport
  Pboost_u/Pboost_r : Inport  Port=2
  Speed_init : Inport  Port=3
  Throttle_init[%] : Inport  Port=4
  Speed : Inport  Port=5
  Throttle_act[%] : Inport  Port=6
  Boost : Subsystem
  Logical Operator : Logic  Operator=NOT  AllPortsSameDT=off  OutDataTypeStr=boolean
  Logical Operator1 : Logic  AllPortsSameDT=off  OutDataTypeStr=boolean
  Memory2 : Memory  X0=1
  Merge : Merge
  Msub : Lookup_n-D  BreakpointsForDimension1=Speed  BreakpointsForDimension2=Pedal  BreakpointsForDimension3=Pedal  Table=Mbu_sub_end  ExtrapMethod=Clip  UseLastTableValue=on  RndMeth=Simplest
  Relational Operator : RelationalOperator  Operator=<=  OutDataTypeStr=boolean
  Subatmo : Subsystem
  dPboost/dt : Lookup_n-D  NumberOfTableDimensions=3  BreakpointsForDimension1=dP  BreakpointsForDimension2=Speed  BreakpointsForDimension3=Pedal  Table=time_dP  ExtrapMethod=Clip  UseLastTableValue=on  RndMeth=Simplest
  BUS_Derivatives : Outport
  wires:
  Speed/1 -> Subatmo/1(Speed), dPboost/dt/2, Boost/2(Speed)
  Speed_init/1 -> Msub/1
  Msub/1 -> Relational Operator/2
  Logical Operator1/1 -> Memory2/1, Logical Operator/1, Subatmo/Enable
  Mbu/1 -> Relational Operator/1
  Logical Operator/1 -> Boost/Enable
  dPboost/dt/1 -> Boost/1(Timer)
  Memory2/1 -> Logical Operator1/2
  Relational Operator/1 -> Logical Operator1/1
  Boost/1(BUS_derivatives_boost) -> Merge/2
  Pboost_u/Pboost_r/1 -> dPboost/dt/1
  Throttle_init[%]/1 -> Boost/3(Throttle[%]), Subatmo/2(Throttle), Msub/2, dPboost/dt/3
  Subatmo/1(BUS_derivatives_sub) -> Merge/1
  Merge/1 -> BUS_Derivatives/1
  Throttle_act[%]/1 -> Subatmo/3(Throttle_act[%])

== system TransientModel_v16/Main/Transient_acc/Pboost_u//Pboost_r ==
  Pboost_u : Inport
  Pboostr_max[bar] : Inport  Port=2
  Pboost_init : Inport  Port=3
  Add : Sum  Inputs=+-
  Add1 : Sum  Inputs=+-
  Divide : Product  Inputs=*/
  Mux : Mux  Inputs=2
  Mux1 : Mux  Inputs=2
  Saturation : Saturate  UpperLimit=1  LowerLimit=0
  Scope : Scope  NumInputPorts=3
  Pboost_u/Pboost_r : Outport
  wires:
  Divide/1 -> Saturation/1
  Pboost_u/1 -> Mux/1, Add/1
  Pboost_init/1 -> Mux1/2, Mux/2, Add/2, Add1/2
  Add/1 -> Divide/1
  Add1/1 -> Divide/2
  Pboostr_max[bar]/1 -> Mux1/1, Add1/1
  Saturation/1 -> Scope/3, Pboost_u/Pboost_r/1
  Mux/1 -> Scope/1
  Mux1/1 -> Scope/2

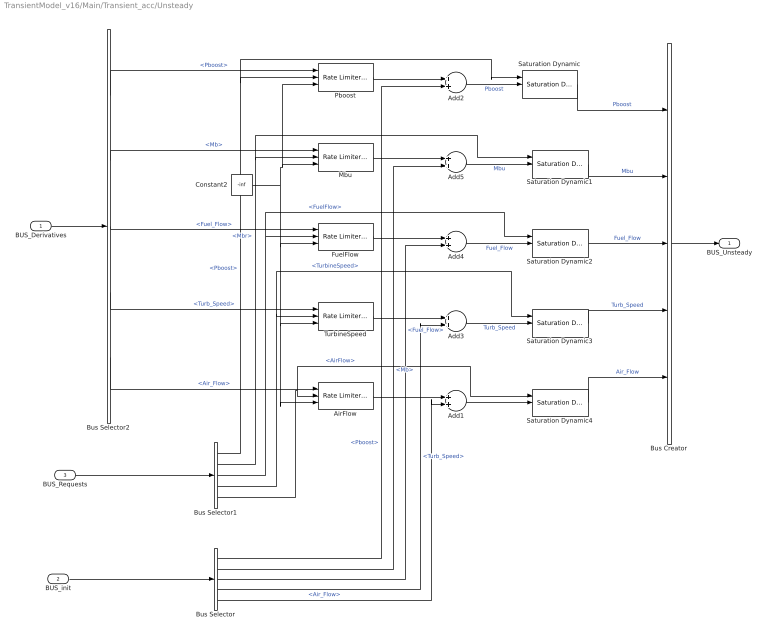
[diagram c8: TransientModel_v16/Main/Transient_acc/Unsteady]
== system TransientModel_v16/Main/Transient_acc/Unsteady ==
  BUS_Derivatives : Inport
  BUS_init : Inport  Port=2
  BUS_Requests : Inport  Port=3
  Add{1..5} (5 alike) : Sum
  AirFlow : simulink/Discontinuities/Rate Limiter Dynamic
  Bus Creator : BusCreator  Inputs=5
  Bus Selector : BusSelector  OutputSignals=Pboost,Mb,Fuel_Flow,Turb_Speed,Air_Flow
  Bus Selector1 : BusSelector  OutputSignals=Pboost,Mbr,FuelFlow,TurbineSpeed,AirFlow
  Bus Selector2 : BusSelector  OutputSignals=Pboost,Mb,Fuel_Flow,Turb_Speed,Air_Flow
  Constant2 : Constant  Value=-inf
  FuelFlow : simulink/Discontinuities/Rate Limiter Dynamic
  Mbu : simulink/Discontinuities/Rate Limiter Dynamic
  Pboost : simulink/Discontinuities/Rate Limiter Dynamic
  Saturation Dynamic{,1..4} (5 alike) : simulink/Discontinuities/Saturation Dynamic  OutMin=[]  OutMax=[]  OutDataTypeStr=Inherit: Same as second input  OutDataType=fixdt(1, 16)  OutScaling=2^-10  DoSatur=off
  TurbineSpeed : simulink/Discontinuities/Rate Limiter Dynamic
  BUS_Unsteady : Outport
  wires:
  Bus Selector2/4 -> TurbineSpeed/1  "<Turb_Speed>"
  Bus Selector2/2 -> Mbu/1  "<Mb>"
  Bus Selector2/3 -> FuelFlow/1  "<Fuel_Flow>"
  Bus Selector2/1 -> Pboost/1  "<Pboost>"
  Bus Selector/2 -> Add5/2  "<Mb>"
  Bus Selector/3 -> Add4/2  "<Fuel_Flow>"
  Bus Selector/4 -> Add3/2  "<Turb_Speed>"
  Constant2/1 -> Pboost/3, Mbu/3, AirFlow/3, TurbineSpeed/3, FuelFlow/3
  TurbineSpeed/1 -> Add3/1
  BUS_init/1 -> Bus Selector/1
  BUS_Derivatives/1 -> Bus Selector2/1
  Mbu/1 -> Add5/1
  FuelFlow/1 -> Add4/1
  BUS_Requests/1 -> Bus Selector1/1
  Bus Selector1/3 -> FuelFlow/2, Saturation Dynamic2/1  "<FuelFlow>"
  Bus Selector1/4 -> TurbineSpeed/2, Saturation Dynamic3/1  "<TurbineSpeed>"
  Bus Creator/1 -> BUS_Unsteady/1
  Pboost/1 -> Add2/1
  Bus Selector/1 -> Add2/2  "<Pboost>"
  Bus Selector1/1 -> Saturation Dynamic/1, Pboost/2  "<Pboost>"
  Bus Selector1/2 -> Mbu/2, Saturation Dynamic1/1  "<Mbr>"
  Add2/1 -> Saturation Dynamic/2  "Pboost"
  Saturation Dynamic/1 -> Bus Creator/1  "Pboost"
  Add5/1 -> Saturation Dynamic1/2  "Mbu"
  Saturation Dynamic1/1 -> Bus Creator/2  "Mbu"
  Add4/1 -> Saturation Dynamic2/2  "Fuel_Flow"
  Saturation Dynamic2/1 -> Bus Creator/3  "Fuel_Flow"
  Add3/1 -> Saturation Dynamic3/2  "Turb_Speed"
  Saturation Dynamic3/1 -> Bus Creator/4  "Turb_Speed"
  Bus Selector2/5 -> AirFlow/1  "<Air_Flow>"
  Bus Selector1/5 -> Saturation Dynamic4/1, AirFlow/2  "<AirFlow>"
  AirFlow/1 -> Add1/1
  Add1/1 -> Saturation Dynamic4/2
  Saturation Dynamic4/1 -> Bus Creator/5  "Air_Flow"
  Bus Selector/5 -> Add1/2  "<Air_Flow>"

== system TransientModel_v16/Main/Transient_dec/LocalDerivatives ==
  Pboost_u/Pboost_r : Inport
  Speed_init : Inport  Port=2
  Speed : Inport  Port=3
  Boost : Subsystem
  dPboost/dt : Lookup_n-D  BreakpointsForDimension1=dP_drag  BreakpointsForDimension2=Speed  BreakpointsForDimension3=Pedal  Table=time_dP_drag  ExtrapMethod=Clip  UseLastTableValue=on  RndMeth=Simplest
  BUS_Derivatives : Outport
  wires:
  Boost/1(BUS_derivatives_boost) -> BUS_Derivatives/1
  Pboost_u/Pboost_r/1 -> dPboost/dt/1
  dPboost/dt/1 -> Boost/1(Timer)
  Speed_init/1 -> dPboost/dt/2
  Speed/1 -> Boost/2(Speed)

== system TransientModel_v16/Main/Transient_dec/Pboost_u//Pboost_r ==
  Pboost_u : Inport
  Pboostr_max[bar] : Inport  Port=2
  Pboost_init : Inport  Port=3
  Add : Sum  Inputs=-+
  Add1 : Sum  Inputs=+-
  Add2 : Sum  Inputs=+-
  Constant : Constant
  Divide : Product  Inputs=*/
  Saturation : Saturate  UpperLimit=1  LowerLimit=0
  Pboost_u/Pboost_r : Outport
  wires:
  Pboostr_max[bar]/1 -> Add/2, Add1/1
  Pboost_init/1 -> Add1/2
  Pboost_u/1 -> Add/1
  Add1/1 -> Divide/2
  Add/1 -> Divide/1
  Saturation/1 -> Pboost_u/Pboost_r/1
  Constant/1 -> Add2/1
  Add2/1 -> Saturation/1
  Divide/1 -> Add2/2

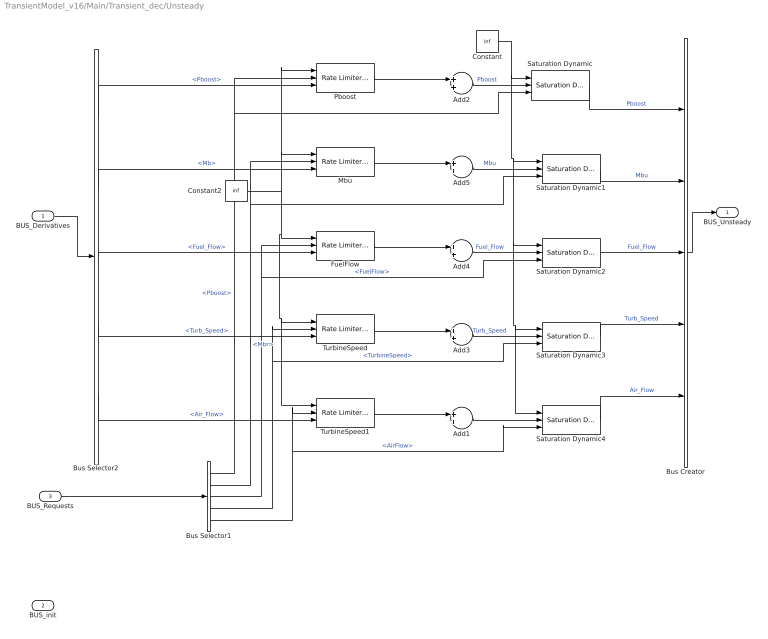
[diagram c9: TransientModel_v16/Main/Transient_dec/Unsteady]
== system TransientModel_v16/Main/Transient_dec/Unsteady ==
  BUS_Derivatives : Inport
  BUS_init : Inport  Port=2
  BUS_Requests : Inport  Port=3
  Add{1..5} (5 alike) : Sum
  Bus Creator : BusCreator  Inputs=5
  Bus Selector1 : BusSelector  OutputSignals=Pboost,Mbr,FuelFlow,TurbineSpeed,AirFlow
  Bus Selector2 : BusSelector  OutputSignals=Pboost,Mb,Fuel_Flow,Turb_Speed,Air_Flow
  Constant : Constant  Value=inf
  Constant2 : Constant  Value=inf
  FuelFlow : simulink/Discontinuities/Rate Limiter Dynamic
  Mbu : simulink/Discontinuities/Rate Limiter Dynamic
  Pboost : simulink/Discontinuities/Rate Limiter Dynamic
  Saturation Dynamic{,1..4} (5 alike) : simulink/Discontinuities/Saturation Dynamic  OutMin=[]  OutMax=[]  OutDataTypeStr=Inherit: Same as second input  OutDataType=fixdt(1, 16)  OutScaling=2^-10  DoSatur=off
  TurbineSpeed : simulink/Discontinuities/Rate Limiter Dynamic
  TurbineSpeed1 : simulink/Discontinuities/Rate Limiter Dynamic
  BUS_Unsteady : Outport
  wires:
  Saturation Dynamic3/1 -> Bus Creator/4  "Turb_Speed"
  Add3/1 -> Saturation Dynamic3/2  "Turb_Speed"
  Saturation Dynamic2/1 -> Bus Creator/3  "Fuel_Flow"
  Add4/1 -> Saturation Dynamic2/2  "Fuel_Flow"
  Saturation Dynamic1/1 -> Bus Creator/2  "Mbu"
  Add5/1 -> Saturation Dynamic1/2  "Mbu"
  Saturation Dynamic/1 -> Bus Creator/1  "Pboost"
  Add2/1 -> Saturation Dynamic/2  "Pboost"
  Bus Selector1/2 -> Saturation Dynamic1/3, Mbu/2  "<Mbr>"
  Bus Selector1/1 -> Saturation Dynamic/3, Pboost/2  "<Pboost>"
  Pboost/1 -> Add2/1
  Bus Creator/1 -> BUS_Unsteady/1
  Bus Selector1/4 -> Saturation Dynamic3/3, TurbineSpeed/2  "<TurbineSpeed>"
  Bus Selector1/3 -> FuelFlow/2, Saturation Dynamic2/3  "<FuelFlow>"
  BUS_Requests/1 -> Bus Selector1/1
  FuelFlow/1 -> Add4/1
  Mbu/1 -> Add5/1
  BUS_Derivatives/1 -> Bus Selector2/1
  BUS_init/1 -> ?
  TurbineSpeed/1 -> Add3/1
  Bus Selector2/1 -> Pboost/3  "<Pboost>"
  Bus Selector2/2 -> Mbu/3  "<Mb>"
  Bus Selector2/3 -> FuelFlow/3  "<Fuel_Flow>"
  Bus Selector2/4 -> TurbineSpeed/3  "<Turb_Speed>"
  Constant2/1 -> TurbineSpeed1/1, TurbineSpeed/1, FuelFlow/1, Pboost/1, Mbu/1
  Constant/1 -> Saturation Dynamic4/1, Saturation Dynamic3/1, Saturation Dynamic2/1, Saturation Dynamic1/1, Saturation Dynamic/1
  Bus Selector2/5 -> TurbineSpeed1/3  "<Air_Flow>"
  Bus Selector1/5 -> Saturation Dynamic4/3, TurbineSpeed1/2  "<AirFlow>"
  TurbineSpeed1/1 -> Add1/1
  Add1/1 -> Saturation Dynamic4/2
  Saturation Dynamic4/1 -> Bus Creator/5  "Air_Flow"

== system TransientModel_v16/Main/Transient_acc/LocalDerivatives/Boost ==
  Timer : Inport
  Speed : Inport  Port=2
  Throttle[%] : Inport  Port=3
  Enable : EnablePort  StatesWhenEnabling=reset
  Bus Creator : BusCreator  Inputs=5
  Gain{,1..4} (5 alike) : Gain
  dMbu/dt : Lookup_n-D  NumberOfTableDimensions=3  BreakpointsForDimension1=time_dy  BreakpointsForDimension2=Speed  BreakpointsForDimension3=Pedal  Table=dY_Mbu  ExtrapMethod=Clip  UseLastTableValue=on  RndMeth=Simplest
  dMbu/dt1 : Lookup_n-D  NumberOfTableDimensions=3  BreakpointsForDimension1=time_dy  BreakpointsForDimension2=Speed  BreakpointsForDimension3=Pedal  Table=dY_mf  ExtrapMethod=Clip  UseLastTableValue=on  RndMeth=Simplest
  dMbu/dt2 : Lookup_n-D  NumberOfTableDimensions=3  BreakpointsForDimension1=time_dy  BreakpointsForDimension2=Speed  BreakpointsForDimension3=Pedal  Table=dY_Speed_Turb  ExtrapMethod=Clip  UseLastTableValue=on  RndMeth=Simplest
  dPboost/dt : Lookup_n-D  NumberOfTableDimensions=3  BreakpointsForDimension1=time_dy  BreakpointsForDimension2=Speed  BreakpointsForDimension3=Pedal  Table=dY  ExtrapMethod=Clip  UseLastTableValue=on  RndMeth=Simplest
  daf/dt : Lookup_n-D  NumberOfTableDimensions=3  BreakpointsForDimension1=time_dy  BreakpointsForDimension2=Speed  BreakpointsForDimension3=Pedal  Table=dY_af  ExtrapMethod=Clip  UseLastTableValue=on  RndMeth=Simplest
  BUS_derivatives_boost : Outport
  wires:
  Speed/1 -> dPboost/dt/2, daf/dt/2, dMbu/dt2/2, dMbu/dt1/2, dMbu/dt/2
  Throttle[%]/1 -> dPboost/dt/3, daf/dt/3, dMbu/dt2/3, dMbu/dt1/3, dMbu/dt/3
  Timer/1 -> daf/dt/1, dMbu/dt2/1, dMbu/dt1/1, dMbu/dt/1, dPboost/dt/1
  Gain1/1 -> Bus Creator/1  "Pboost"
  Gain/1 -> Bus Creator/2  "Mb"
  Gain2/1 -> Bus Creator/3  "Fuel_Flow"
  Gain3/1 -> Bus Creator/4  "Turb_Speed"
  Bus Creator/1 -> BUS_derivatives_boost/1
  dPboost/dt/1 -> Gain1/1
  dMbu/dt/1 -> Gain/1
  dMbu/dt2/1 -> Gain3/1
  dMbu/dt1/1 -> Gain2/1
  daf/dt/1 -> Gain4/1
  Gain4/1 -> Bus Creator/5  "Air_Flow"
